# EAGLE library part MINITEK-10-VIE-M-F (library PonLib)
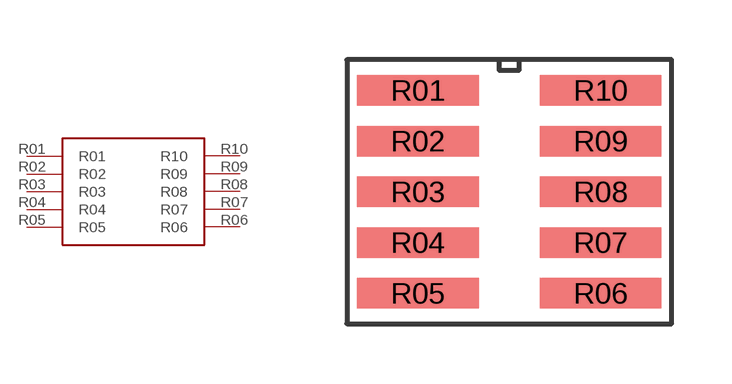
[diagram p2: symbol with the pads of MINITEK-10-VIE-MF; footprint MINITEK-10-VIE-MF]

Designator prefix -

## MINITEK-10-VIE-M-F  [MINITEK-10-VIE-MF]
R01  R01
R02  R02
R03  R03
R04  R04
R05  R05
R06  R06
R07  R07
R08  R08
R09  R09
R10  R10

## Footprint MINITEK-10-VIE-MF (pad centres in mm)
smd 3.048 x 0.762: R01 -2.286,2.54; R02 -2.286,1.27; R03 -2.286,0; R04 -2.286,-1.27; R05 -2.286,-2.54; R06 2.286,-2.54; R07 2.286,-1.27; R08 2.286,0; R09 2.286,1.27; R10 2.286,2.54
